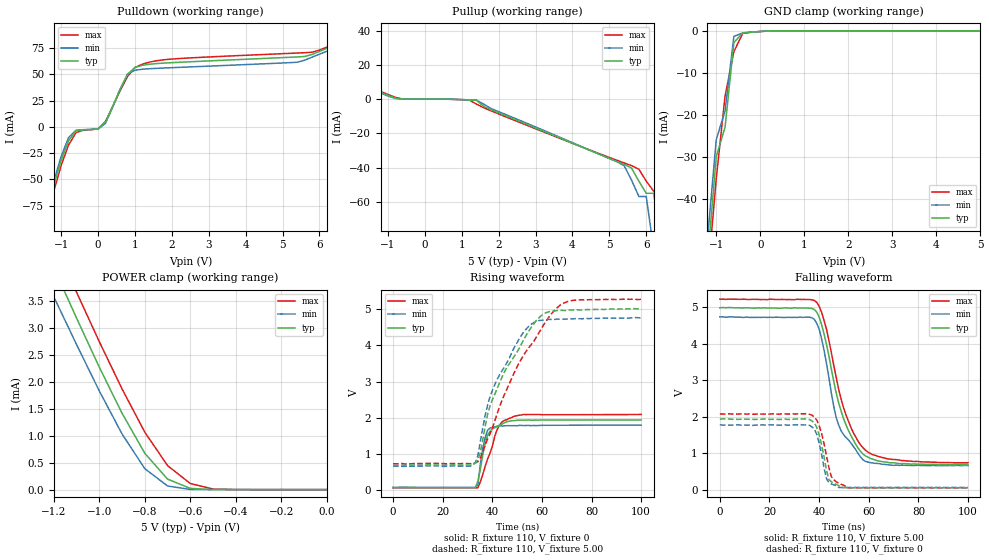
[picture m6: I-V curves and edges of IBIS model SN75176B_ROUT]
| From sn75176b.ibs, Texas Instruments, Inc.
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|   Model SN75176B_ROUT
[Model]   SN75176B_ROUT
Model_type  Output
Polarity   Non-Inverting
Enable   Active-Low
| variable   typ   min   max
C_comp   5.748pf   5.384pf   6.911pf
[Temperature Range]   40   0   85
| Ambient temperature   25   0   70
[Voltage Range]   5.00   4.75   5.25
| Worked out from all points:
|   slope of the pulldown table from 0 to 0.75 V, typ, clamps not added: 15.4 ohm
|   slope of the pullup table from 0 to 0.75 V, typ, clamps not added: 9.38 kohm
|   GND clamp passes 1 mA (typ) near -0.44 V on its own axis
|   POWER clamp passes 1 mA (typ) near -0.84 V on its own axis
|   rising waveform, R_fixture 110, V_fixture 0: 20-80 % time 3.76ns typ, 2.48ns min, 5.71ns max; typ from 0.058 V to 1.93 V
|   falling waveform, R_fixture 110, V_fixture 5.00: 20-80 % time 9.9ns typ, 8.6ns min, 10.1ns max; typ from 4.98 V to 0.685 V
|   rising waveform, R_fixture 110, V_fixture 5.00: 20-80 % time 16ns typ, 13.3ns min, 19.4ns max; typ from 0.675 V to 5.01 V
|   falling waveform, R_fixture 110, V_fixture 0: 20-80 % time 3.6ns typ, 3.25ns min, 4.13ns max; typ from 1.93 V to 0.058 V
[Pulldown]
|   Voltage   I(typ)   I(min)   I(max)
-5V       -731.1mA   -765.5mA   -678.2mA
-1.6V     -115mA     -113.1mA   -116mA
-1.4V     -83.2mA    -79.43mA   -86.64mA
-1V       -31.54mA   -27.95mA   -36.55mA
-800mV    -13.08mA   -10.04mA   -17.18mA
-600mV    -3.801mA   -3.13mA    -5.418mA
200mV     4.424mA    3.389mA    5.162mA
800mV     50.25mA    50.36mA    48.2mA
1.2V      58.68mA    54.97mA    59.8mA
5.4V      66.67mA    61.62mA    70.38mA
7.8V      97.42mA    94.29mA    98.28mA
10V       128.4mA    125.2mA    128.5mA
[Pullup]
|   Voltage   I(typ)   I(min)   I(max)
-5V       40.84mA    39.65mA    41.53mA
-800mV    676.6uA    398uA      1.053mA
1.4V      -690.1uA   -563.3uA   -2.904mA
5.2V      -36.34mA   -36.57mA   -35.69mA
5.4V      -38.07mA   -38.83mA   -37.28mA
5.6V      -40.24mA   -47.29mA   -38.86mA
5.8V      -47.99mA   -56.91mA   -40.96mA
6V        -55.04mA   -56.91mA   -47.95mA
6.2V      -55.04mA   -87.78mA   -53.76mA
6.4V      -83.52mA   -122.3mA   -53.76mA
6.6V      -115.3mA   -158.7mA   -79.62mA
10V       -727.4mA   -813.9mA   -639.1mA
[GND Clamp]
|   Voltage   I(typ)   I(min)   I(max)
-5V       -728.6mA   -765.7mA   -678.2mA
-1.2V     -54.85mA   -49.71mA   -59.45mA
-1V       -29.98mA   -25.93mA   -35.23mA
-800mV    -22.96mA   -19.04mA   -15.55mA
-600mV    -2.802mA   -1.33mA    -4.989mA
-400mV    -501.9uA   -497.4uA   -614.5uA
-200mV    -324.2uA   -324.4uA   -318uA
400mV     -52.46nA   -16.85nA   -153nA
5V        73.9pA     7.7pA      2.507nA
[POWER Clamp]
|   Voltage   I(typ)   I(min)   I(max)
-5V       40.88mA    39.61mA    41.51mA
-1.2V     4.112mA    3.574mA    4.601mA
-1.1V     3.18mA     2.689mA    3.659mA
-1V       2.269mA    1.829mA    2.742mA
-900mV    1.415mA    1.031mA    1.866mA
-800mV    673.1uA    388uA      1.064mA
-700mV    194.4uA    67.18uA    444.5uA
-600mV    22.49uA    2.547uA    112.6uA
-500mV    714.5nA    43.74nA    11.06uA
9.77fV    73.9pA     3.8pA      2.159nA
[Ramp]
| variable   typ   min   max
dV/dt_r  1.104E+00/3.783E-09  9.960E-01/2.572E-09  1.194E+00/1.235E-08
dV/dt_f  2.634E+00/1.009E-08  2.496E+00/1.005E-08  2.736E+00/1.041E-08
R_load = 110
[Rising Waveform]
R_fixture = 110
V_fixture = 0
V_fixture_min = 0
V_fixture_max = 0
C_fixture = 0pf
L_fixture = 0nH
|   Time   V(typ)   V(min)   V(max)
0s        58.27mV    65.3mV     53.64mV
33.2ns    58.26mV    66.42mV    51.44mV
34.18ns   238.3mV    129.7mV    52.34mV
35.16ns   559.1mV    708.8mV    213.6mV
36.13ns   953.7mV    1.134V     415.2mV
38.09ns   1.51V      1.646V     848.4mV
41.02ns   1.721V     1.743V     1.493V
42.97ns   1.796V     1.775V     1.8V
48.83ns   1.914V     1.776V     2.039V
100ns     1.934V     1.79V      2.085V
[Falling Waveform]
R_fixture = 110
V_fixture = 5.00
V_fixture_min = 4.75
V_fixture_max = 5.25
C_fixture = 0pf
L_fixture = 0nH
|   Time   V(typ)   V(min)   V(max)
0s        4.977V     4.727V     5.212V
38.09ns   4.929V     4.658V     5.174V
40.04ns   4.716V     4.387V     5.015V
42.97ns   3.972V     3.455V     4.391V
45.9ns    2.967V     2.278V     3.401V
47.85ns   2.381V     1.778V     2.753V
51.76ns   1.626V     1.368V     1.881V
57.62ns   981.8mV    824mV      1.155V
68.36ns   740.5mV    681.9mV    840.2mV
100ns     684.7mV    663.3mV    743.3mV
[Rising Waveform]
R_fixture = 110
V_fixture = 5.00
V_fixture_min = 4.75
V_fixture_max = 5.25
C_fixture = 0pf
L_fixture = 0nH
|   Time   V(typ)   V(min)   V(max)
0s        674.9mV    653.1mV    717.2mV
33.2ns    736.4mV    760.7mV    746.6mV
35.16ns   1.027V     1.331V     872.1mV
38.09ns   2.093V     2.344V     1.402V
41.02ns   2.652V     2.918V     1.909V
49.8ns    3.799V     4.054V     3.382V
56.64ns   4.587V     4.632V     4.106V
63.48ns   4.944V     4.723V     4.85V
70.31ns   4.98V      4.735V     5.217V
100ns     5.012V     4.77V      5.281V
[Falling Waveform]
R_fixture = 110
V_fixture = 0
V_fixture_min = 0
V_fixture_max = 0
C_fixture = 0pf
L_fixture = 0nH
|   Time   V(typ)   V(min)   V(max)
0s        1.932V     1.775V     2.076V
37.11ns   1.883V     1.72V      2.04V
39.06ns   1.701V     1.51V      1.903V
40.04ns   1.499V     1.271V     1.75V
42.97ns   535.1mV    307.9mV    933.1mV
43.95ns   279.4mV    196.1mV    604.1mV
44.92ns   223.5mV    160.1mV    362.1mV
45.9ns    177.9mV    136mV      277mV
51.76ns   58.69mV    65.18mV    54.19mV
100ns     58.17mV    65.29mV    54.24mV
